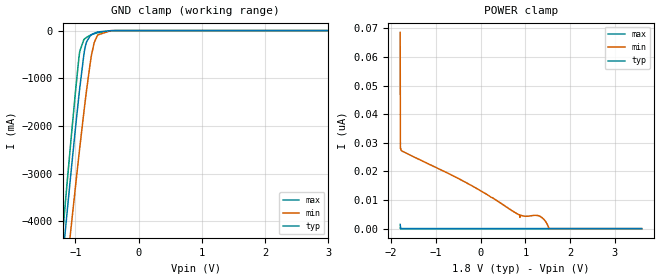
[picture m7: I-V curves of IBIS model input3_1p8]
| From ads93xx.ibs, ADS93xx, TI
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|   input3_1p8 Model
[Model]   input3_1p8
Model_type   Input
Vinl = 0.5
Vinh = 1.3
|   typ   min   max
C_comp   5.077pF   4.893pF   5.244pF
[Voltage Range]   1.8   1.65   1.95
[Temperature Range]   27   125   -40
[Power Clamp Reference]   1.8   1.65   1.95
[GND Clamp Reference]   0   0   0
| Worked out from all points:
|   GND clamp passes 1 mA (typ) near -0.41 V on its own axis
[GND Clamp]
|   Voltage   I(typ)   I(min)   I(max)
-1.8V     -12.26A    -11.59A    -13.13A
-1.39V    -7.407A    -8.137A    -7.12A
-1.147V   -4.011A    -5.109A    -3.416A
-1.071V   -2.984A    -4.156A    -2.3A
-995.4mV  -1.992A    -3.222A    -1.228A
-930.6mV  -1.194A    -2.444A    -429.6mA
-855mV    -407.2mA   -1.584A    -173mA
-768.6mV  -113.4mA   -705.5mA   -99.45mA
-703.8mV  -58.81mA   -255.6mA   -63.9mA
-649.8mV  -29.54mA   -93.3mA    -45.36mA
-444.6mV  -1.862mA   -2.185mA   -5.304mA
3.6V      0A         0A         0A
[POWER Clamp]
|   Voltage   I(typ)   I(min)   I(max)
-1.8V     1.486nA    68.6nA     232.2pA
-1.795V   743.2pA    28.04nA    116.1pA
-1.789V   0A         28.03nA    0A
-1.762V   0A         27.17nA    0A
-136.8mV  0A         14.47nA    0A
862.2mV   0A         4.798nA    0A
878.4mV   0A         3.951nA    0A
883.8mV   0A         4.753nA    0A
1.327V    0A         4.305nA    0A
1.44V     0A         2.747nA    0A
1.537V    0A         0A         0A
3.6V      0A         0A         0A
